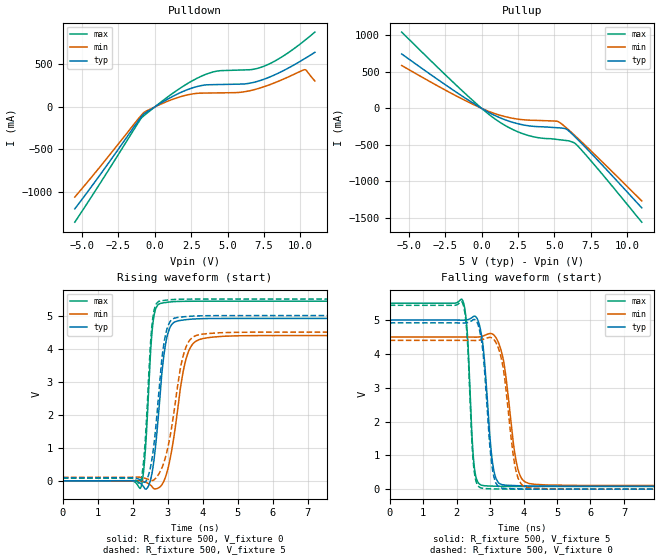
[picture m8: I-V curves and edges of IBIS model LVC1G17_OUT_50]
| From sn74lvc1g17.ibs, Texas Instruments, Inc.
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[Model]   LVC1G17_OUT_50
Model_type  Output
Vref =   0
Rref =   500
Cref =   50p
Vmeas =   2.5
| variable   typ   min   max
C_comp   8.84pF   5.46pF   12.36pF
| C_pullup   9.69pF   5.46pF   12.36pF
| C_pulldown   7.99pF   5.90pF   10.96pF
[Temperature Range]   40   100   -40
| Ambient temperature   25   85   -40
[Voltage range]   5   4.5   5.5
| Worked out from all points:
|   slope of the pulldown table from 0 to 0.75 V, typ, clamps not added: 9.58 ohm
|   slope of the pullup table from 0 to 0.75 V, typ, clamps not added: 9.16 ohm
|   rising waveform, R_fixture 500, V_fixture 0: 20-80 % time 263ps typ, 377ps min, 169ps max; typ from 0 V to 4.91 V
|   falling waveform, R_fixture 500, V_fixture 5: 20-80 % time 227ps typ, 319ps min, 152ps max; typ from 5 V to 0.09 V
|   rising waveform, R_fixture 500, V_fixture 5: 20-80 % time 269ps typ, 405ps min, 172ps max; typ from 0.09 V to 5 V
|   falling waveform, R_fixture 500, V_fixture 0: 20-80 % time 223ps typ, 309ps min, 151ps max; typ from 4.92 V to 0 V
[Pulldown]
| LVC1G17_OUT_50
|   Voltage   I(typ)   I(min)   I(max)
-5.5V     -1.198A    -1.059A    -1.354A
-970mV    -125.1mA   -106.1mA   -141.7mA
-675mV    -74.35mA   -56.48mA   -92.74mA
205mV     22.29mA    16.59mA    27.99mA
1.905V    179.2mA    127mA      238mA
3.285V    253.2mA    162.4mA    367.3mA
4.325V    262.7mA    164.8mA    422.2mA
5.815V    267.8mA    170.7mA    433mA
7.31V     313.8mA    226.4mA    466mA
8.65V     410.1mA    312.7mA    578.8mA
10.28V    565mA      437.4mA    777.7mA
11V       641.2mA    305.2mA    879.1mA
[Pullup]
| LVC1G17_OUT_50
|   Voltage   I(typ)   I(min)   I(max)
-5.5V     745.2mA    587.5mA    1.044A
-1.18V    147.6mA    112.6mA    211.7mA
170mV     -19.98mA   -14.91mA   -29.14mA
1.04V     -109.2mA   -79.97mA   -161.6mA
2.045V    -185.4mA   -131.8mA   -280mA
3.05V     -232.7mA   -158.7mA   -361.3mA
3.945V    -250.5mA   -165.3mA   -402.5mA
5.3V      -265.9mA   -185.4mA   -427.7mA
5.83V     -285.1mA   -268.2mA   -440mA
6.525V    -410.2mA   -394.3mA   -498.1mA
8.085V    -732.8mA   -692.6mA   -852.4mA
11V       -1.361A    -1.267A    -1.557A
[Ramp]
| LVC1G17_OUT_50
| variable   typ   min   max
dV/dt_r   3.10/2.83E-10   2.78/4.08E-10   3.40/1.80E-10
dV/dt_f   3.02/2.40E-10   2.70/3.38E-10   3.33/1.58E-10
R_load = 500
[Rising Waveform]
| LVC1G17_OUT_50
R_fixture =   500
C_fixture =   0
L_fixture =   0
V_fixture =   0
V_fixture_min = 0
V_fixture_max = 0
|   Time   V(typ)   V(min)   V(max)
0s        181.8pV    4.248nV    2.638nV
2.225ns   -81.72mV   -2.134mV   -215.3mV
2.35ns    -243.1mV   -36.84mV   768.9mV
2.57ns    354.6mV    -203.6mV   4.7V
2.805ns   2.889V     -157.4mV   5.371V
2.935ns   4.11V      110.8mV    5.394V
3.09ns    4.693V     781.4mV    5.414V
3.52ns    4.876V     3.671V     5.433V
4.01ns    4.907V     4.306V     5.435V
22.4ns    4.914V     4.397V     5.435V
[Falling Waveform]
| LVC1G17_OUT_50
R_fixture =   500
C_fixture =   0
L_fixture =   0
V_fixture =   5
V_fixture_min = 4.5
V_fixture_max = 5.5
|   Time   V(typ)   V(min)   V(max)
0s        5V         4.5V       5.5V
2.18ns    4.998V     4.5V       5.582V
2.325ns   5.01V      4.5V       4.549V
2.52ns    5.114V     4.497V     733.2mV
2.75ns    4.522V     4.518V     116.2mV
3.075ns   777mV      4.585V     90.43mV
3.365ns   130.7mV    3.966V     83.52mV
3.795ns   103.5mV    748.1mV    80.28mV
4.17ns    94.48mV    165.6mV    79.47mV
22.4ns    89.64mV    107.6mV    78.98mV
[Rising Waveform]
| LVC1G17_OUT_50
R_fixture =   500
C_fixture =   0
L_fixture =   0
V_fixture =   5
V_fixture_min = 4.5
V_fixture_max = 5.5
|   Time   V(typ)   V(min)   V(max)
0s        89.62mV    107.6mV    78.96mV
2.21ns    29.94mV    108.2mV    -72.64mV
2.34ns    -44.54mV   79.52mV    958.8mV
2.555ns   696.1mV    8.655mV    4.764V
2.755ns   2.776V     223.6mV    5.435V
2.89ns    4.145V     551.5mV    5.459V
3.06ns    4.803V     1.303V     5.479V
3.45ns    4.963V     3.811V     5.497V
3.905ns   4.992V     4.423V     5.5V
22.4ns    5V         4.5V       5.5V
[Falling Waveform]
| LVC1G17_OUT_50
R_fixture =   500
C_fixture =   0
L_fixture =   0
V_fixture =   0
V_fixture_min = 0
V_fixture_max = 0
|   Time   V(typ)   V(min)   V(max)
0s        4.917V     4.401V     5.437V
2.175ns   4.915V     4.401V     5.512V
2.32ns    4.926V     4.401V     4.447V
2.51ns    5.016V     4.398V     673.1mV
2.745ns   4.381V     4.418V     30.34mV
3.06ns    664.5mV    4.469V     9.933mV
3.355ns   30.51mV    3.774V     4.069mV
3.76ns    11.65mV    611.1mV    1.29mV
4.145ns   3.993mV    42.49mV    494.7uV
22.4ns    17.3uV     23.17uV    17.91uV
